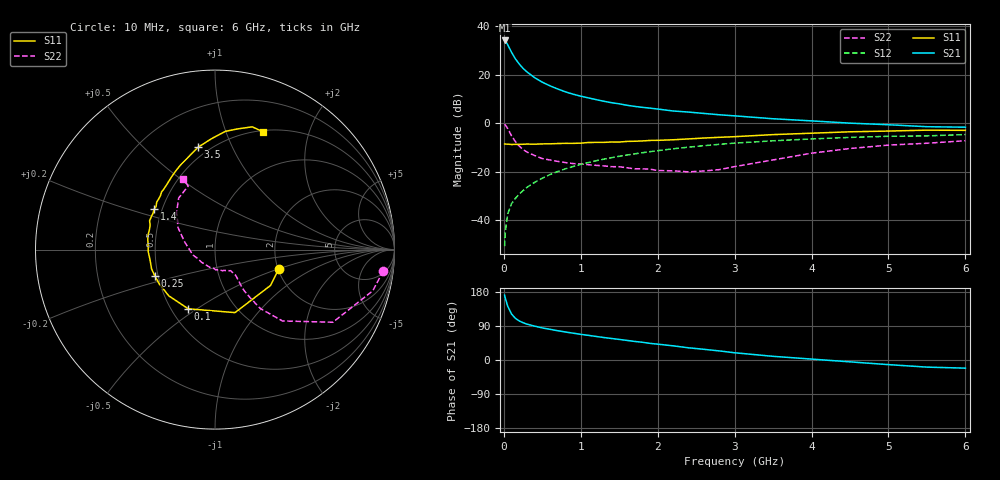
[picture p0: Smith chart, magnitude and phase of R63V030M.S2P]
! SIEMENS Small Signal Semiconductors
! BFR193
! Si NPN RF Bipolar Junction Transistor in SOT23
! VCE = 3 V  IC = 30 mA
! Common Emitter S-Parameters:  May  1996
# GHz  S  MA  R  50
!  f  S11  S21  S12  S22
! GHz  MAG  ANG  MAG  ANG  MAG  ANG  MAG  ANG
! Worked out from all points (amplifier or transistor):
!   36 points, 10 MHz to 6 GHz, reference 50 ohm
!   highest |S21| = 34.1 dB at 10 MHz (marker M1)
!   |S21| within 3 dB of that: start of sweep to 70.24 MHz
!   unconditionally stable (mu >= 1): 460.5 MHz to 1.859 GHz
!   at 250 MHz: K = 0.90, MSG = 25.2 dB, |S12| = -27.9 dB
!   at 1.4 GHz: K = 1.02, MAG = 10.4 dB, |S12| = -14.3 dB
!   at 6 GHz: K = 0.94, MSG = 1.5 dB, |S12| = -4.7 dB
!   lowest NFmin = 1.90 dB at 450 MHz
!   S11 on the Smith chart (normalised r, x): 10 MHz: 2.01, -0.51; 100 MHz: 0.61, -0.46; 250 MHz: 0.48, -0.16; 1.4 GHz: 0.45, +0.25; 3.5 GHz: 0.44, +0.75; 6 GHz: 0.52, +1.36
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0.01  0.3707 -17.1  50.51 171.1  0.0029 82.0  0.9454 -7.2
0.02  0.3684 -32.8  49.2 162.7  0.0059 81.8  0.9087 -14.6
0.05  0.3683 -72.4  41.38 142.1  0.0134 69.4  0.772 -31.6
0.1  0.3619 -114.3  28.85 121.5  0.0218 66.2  0.5473 -46.6
0.15  0.3641 -134.9  21.11 110.0  0.028 65.7  0.4147 -52.4
0.2  0.3648 -148.3  16.53 103.1  0.0344 67.8  0.3359 -53.8
0.25  0.366 -156.6  13.42 98.4  0.0405 68.8  0.2846 -54.6
0.3  0.3693 -162.9  11.36 94.7  0.0473 70.3  0.2533 -54.3
0.4  0.3668 -172.2  8.639 89.4  0.06 71.4  0.2143 -52.8
0.5  0.3722 -178.2  6.967 84.7  0.0731 71.8  0.1852 -51.2
0.6  0.3736 176.3  5.855 81.0  0.0869 71.8  0.1734 -51.7
0.7  0.3789 171.2  5.048 77.2  0.1003 71.2  0.1623 -52.2
0.8  0.382 167.4  4.41 73.9  0.1139 70.3  0.1534 -53.0
0.9  0.3818 163.3  3.943 70.8  0.1273 69.3  0.1463 -53.3
1.1  0.3981 156.3  3.304 65.0  0.1539 67.1  0.1386 -57.8
1.4  0.407 146.2  2.631 56.8  0.1936 63.4  0.1263 -66.2
1.7  0.4223 137.9  2.208 49.0  0.2319 59.3  0.1142 -77.2
2.2  0.4528 126.0  1.776 37.4  0.295 52.1  0.1037 -104.9
3.5  0.5785 99.3  1.228 9.7  0.4311 31.9  0.1739 166.0
4.5  0.6613 85.0  0.997 -4.9  0.507 17.6  0.2993 135.6
5.5  0.7149 73.1  0.842 -18.8  0.5445 3.7  0.3842 112.8
6  0.7086 67.7  0.822 -21.5  0.5802 -0.5  0.4324 114.5
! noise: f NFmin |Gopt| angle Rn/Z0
0.45  1.9  0.4  180  0.09
0.9  1.95  0.43  -173  0.11
1.8  2.4  0.58  -144  0.24
